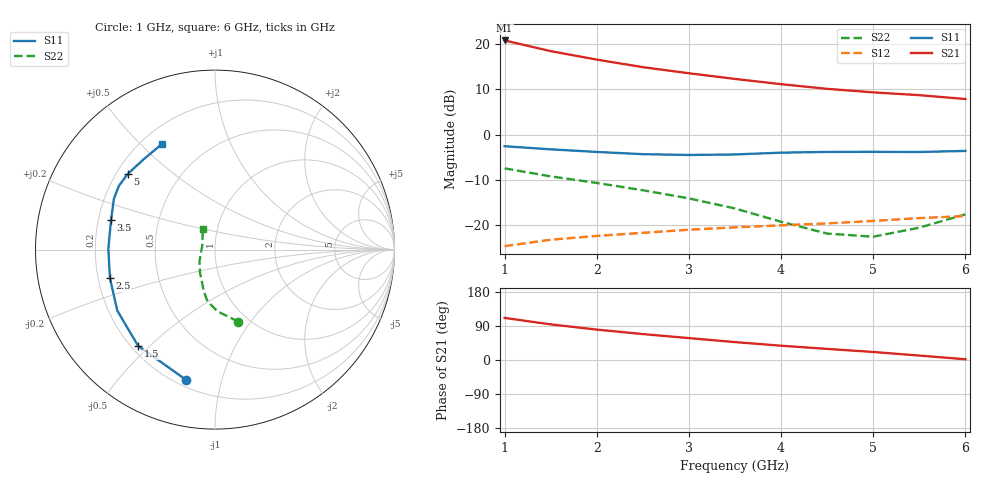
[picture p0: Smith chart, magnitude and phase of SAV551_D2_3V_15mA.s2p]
! Created Mon Oct 27 14:24:35 2008
# hz S ma R 50
! 2 Port Network Data from SP1.SP block
! freq  magS11  angS11  magS21  angS21  magS12  angS12  magS22  angS22
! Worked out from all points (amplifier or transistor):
!   11 points, 1 GHz to 6 GHz, reference 50 ohm
!   highest |S21| = 20.8 dB at 1 GHz (marker M1)
!   |S21| within 3 dB of that: start of sweep to 1.67 GHz
!   unconditionally stable (mu >= 1): 4.36 GHz to end of sweep
!   at 1.5 GHz: K = 0.47, MSG = 20.9 dB, |S12| = -23.3 dB
!   at 3.5 GHz: K = 0.91, MSG = 16.4 dB, |S12| = -20.5 dB
!   at 6 GHz: K = 1.10, MAG = 11.1 dB, |S12| = -18.0 dB
!   S11 on the Smith chart (normalised r, x): 1 GHz: 0.24, -0.77; 1.5 GHz: 0.23, -0.46; 2.5 GHz: 0.25, -0.12; 3.5 GHz: 0.25, +0.13; 5 GHz: 0.25, +0.35; 6 GHz: 0.28, +0.58
1e9  0.7428 -102.6  11 111.0  0.05818 39.5  0.4224 -72.0
1.5e9  0.6862 -128.7  8.376 94.0  0.06856 31.1  0.3445 -87.7
2e9  0.6418 -148.0  6.751 80.2  0.0755 25.2  0.2915 -98.2
2.5e9  0.6065 -164.9  5.567 68.4  0.08172 21.0  0.2419 -104.8
3e9  0.5942 179.5  4.765 57.8  0.08845 17.6  0.1965 -111.5
3.5e9  0.6021 164.2  4.125 47.3  0.09401 13.9  0.152 -123.4
4e9  0.6303 153.3  3.609 37.7  0.09892 10.9  0.1083 -142.7
4.5e9  0.6425 146.4  3.205 29.3  0.104 7.8  0.0802 -167.8
5e9  0.6434 139.2  2.929 21.2  0.1106 4.9  0.07403 163.8
5.5e9  0.6411 128.5  2.727 11.7  0.119 1.4  0.09324 138.4
6e9  0.659 116.5  2.473 2.0  0.1253 -3.5  0.1309 120.8
